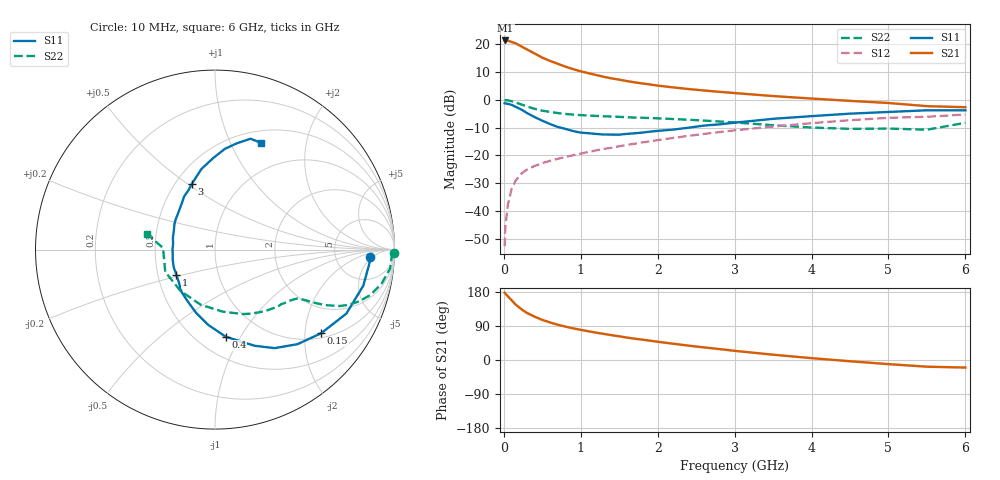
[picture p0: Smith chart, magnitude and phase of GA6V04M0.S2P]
! Infineon Technologies  Discrete & RF Semiconductors
! BF775
! Si NPN RF Bipolar Junction Transistor in SOT23
! VCE = 6 V  IC = 4 mA
! Common Emitter S-Parameters:  May  1996
# GHz  S  MA  R  50
!  f  S11  S21  S12  S22
! GHz  MAG  ANG  MAG  ANG  MAG  ANG  MAG  ANG
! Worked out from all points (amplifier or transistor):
!   36 points, 10 MHz to 6 GHz, reference 50 ohm
!   highest |S21| = 21.4 dB at 20 MHz (marker M1)
!   |S21| within 3 dB of that: start of sweep to 284.8 MHz
!   unconditionally stable (mu >= 1): 899 MHz to 3.176 GHz
!   at 250 MHz: K = 0.41, MSG = 22.5 dB, |S12| = -26.1 dB
!   at 1.4 GHz: K = 1.11, MAG = 10.4 dB, |S12| = -17.3 dB
!   at 6 GHz: K = 0.93, MSG = 1.3 dB, |S12| = -5.3 dB
!   S11 on the Smith chart (normalised r, x): 10 MHz: 13, -4; 150 MHz: 1.13, -2.42; 400 MHz: 0.68, -0.87; 1 GHz: 0.62, -0.19; 3 GHz: 0.60, +0.52; 6 GHz: 0.64, +1.31
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0.01  0.8672 -2.8  11.65 177.6  0.0023 87.1  0.9953 -1.1
0.02  0.8624 -5.6  11.78 175.0  0.005 91.4  0.9849 -2.4
0.05  0.8503 -13.7  11.69 168.5  0.0124 82.2  0.9815 -6.1
0.1  0.814 -26.0  11.1 157.9  0.0244 75.8  0.9477 -11.5
0.15  0.7527 -38.3  10.51 147.0  0.0343 70.0  0.9019 -16.3
0.2  0.6993 -48.9  9.673 138.6  0.0424 65.7  0.8523 -19.8
0.25  0.6417 -58.8  8.838 131.0  0.0495 62.2  0.8052 -22.5
0.3  0.5796 -67.6  8.135 124.3  0.0552 60.0  0.7611 -24.4
0.4  0.4892 -83.0  6.853 114.3  0.0643 56.7  0.6887 -26.7
0.5  0.4204 -95.3  5.775 105.8  0.0723 55.1  0.6386 -27.9
0.6  0.3667 -106.9  5.042 99.1  0.0796 54.7  0.6053 -28.7
0.7  0.3249 -118.2  4.474 93.2  0.0863 55.1  0.5788 -29.2
0.8  0.2998 -128.6  3.975 88.1  0.0934 55.1  0.5582 -29.8
1  0.2568 -146.8  3.271 79.5  0.1076 56.1  0.5306 -31.0
1.1  0.2503 -156.5  3.025 75.8  0.1152 56.1  0.5211 -32.1
1.6  0.2436 164.5  2.181 59.1  0.1536 56.5  0.4867 -37.9
2.2  0.2909 134.4  1.679 43.0  0.2059 54.7  0.4513 -47.7
3  0.3882 109.4  1.327 24.2  0.282 48.5  0.3914 -66.5
3.5  0.4552 99.6  1.171 14.0  0.3301 43.4  0.3487 -82.8
4.5  0.5641 84.4  0.959 -3.3  0.4302 31.2  0.3 -129.9
5.5  0.6487 72.2  0.77 -17.7  0.4957 15.8  0.2894 178.2
6  0.6476 66.7  0.737 -19.9  0.5456 11.5  0.3859 167.3
